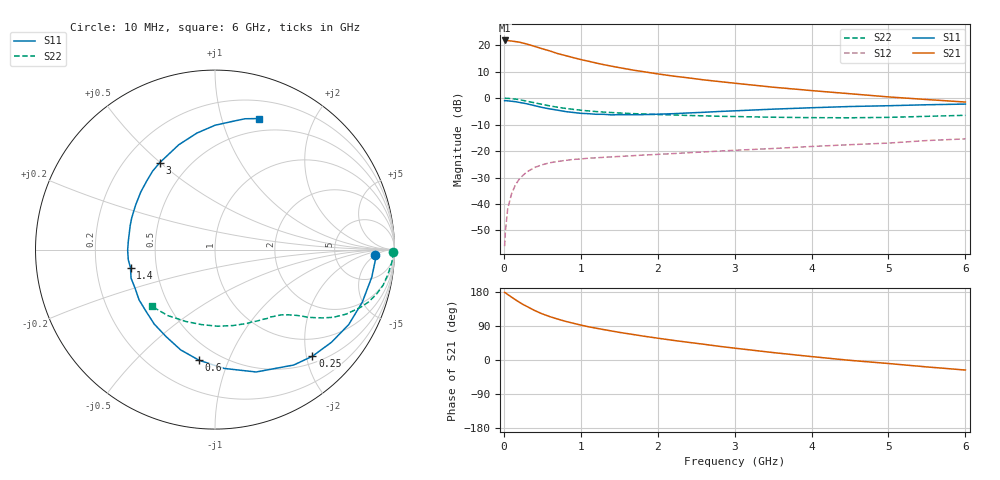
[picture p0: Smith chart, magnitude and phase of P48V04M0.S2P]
! SIEMENS Small Signal Semiconductors
! BFP182
! Si NPN RF Bipolar Junction Transistor in SOT143
! VCE = 8 V  IC = 4 mA
! Common Emitter S-Parameters:  March  1996
# GHz  S  MA  R  50
!  f  S11  S21  S12  S22
! GHz  MAG  ANG  MAG  ANG  MAG  ANG  MAG  ANG
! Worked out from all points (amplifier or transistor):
!   36 points, 10 MHz to 6 GHz, reference 50 ohm
!   highest |S21| = 21.8 dB at 10 MHz (marker M1)
!   |S21| within 3 dB of that: start of sweep to 484.9 MHz
!   unconditionally stable (mu >= 1): 1.822 GHz to 5.746 GHz
!   at 250 MHz: K = 0.18, MSG = 24.9 dB, |S12| = -29.1 dB
!   at 1.4 GHz: K = 0.85, MSG = 17.1 dB, |S12| = -22.2 dB
!   at 6 GHz: K = 0.97, MSG = 7.0 dB, |S12| = -15.4 dB
!   S11 on the Smith chart (normalised r, x): 10 MHz: 16, -5; 250 MHz: 0.63, -2.11; 600 MHz: 0.39, -0.79; 1.4 GHz: 0.35, -0.09; 3 GHz: 0.34, +0.50; 6 GHz: 0.37, +1.33
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0.01  0.8921 -1.9  12.24 178.5  0.0016 79.9  0.9913 -0.8
0.02  0.8949 -3.9  12.18 177.5  0.003 85.6  0.9922 -1.6
0.05  0.887 -9.9  12.15 172.9  0.0081 86.5  0.9878 -4.1
0.1  0.8713 -19.7  11.95 166.0  0.0155 77.7  0.9737 -8.1
0.2  0.8293 -38.5  11.38 152.6  0.0295 68.8  0.9328 -15.5
0.25  0.8047 -47.6  10.91 146.5  0.0349 64.6  0.9031 -18.9
0.3  0.7784 -55.7  10.46 141.3  0.0404 60.7  0.8728 -21.6
0.4  0.7194 -71.4  9.463 130.6  0.0489 53.4  0.8143 -26.2
0.5  0.664 -85.6  8.528 121.7  0.0552 47.9  0.7592 -29.8
0.6  0.6233 -98.1  7.743 114.3  0.0602 43.8  0.71 -32.4
0.7  0.5906 -108.9  6.917 108.0  0.0636 40.4  0.6713 -34.4
0.8  0.5567 -119.1  6.344 102.1  0.0665 37.9  0.6392 -36.1
1  0.5154 -138.3  5.334 92.2  0.0709 34.1  0.5905 -38.5
1.1  0.5074 -146.5  4.96 87.7  0.0733 33.1  0.5716 -39.7
1.4  0.4816 -167.8  4.001 76.6  0.0776 30.4  0.5336 -43.0
1.8  0.4864 168.9  3.179 63.4  0.0838 29.0  0.5017 -47.5
2.2  0.507 150.8  2.603 51.9  0.0895 28.2  0.4806 -53.1
3  0.574 122.4  1.909 31.3  0.1033 26.7  0.4483 -66.7
3.5  0.6179 109.1  1.605 19.6  0.1116 25.2  0.4348 -76.7
4.5  0.6928 90.0  1.207 -0.9  0.1318 21.9  0.4247 -100.4
5.5  0.7478 77.1  0.938 -18.3  0.1578 18.0  0.4521 -125.6
6  0.7704 71.4  0.841 -26.5  0.1697 14.4  0.4727 -138.0
